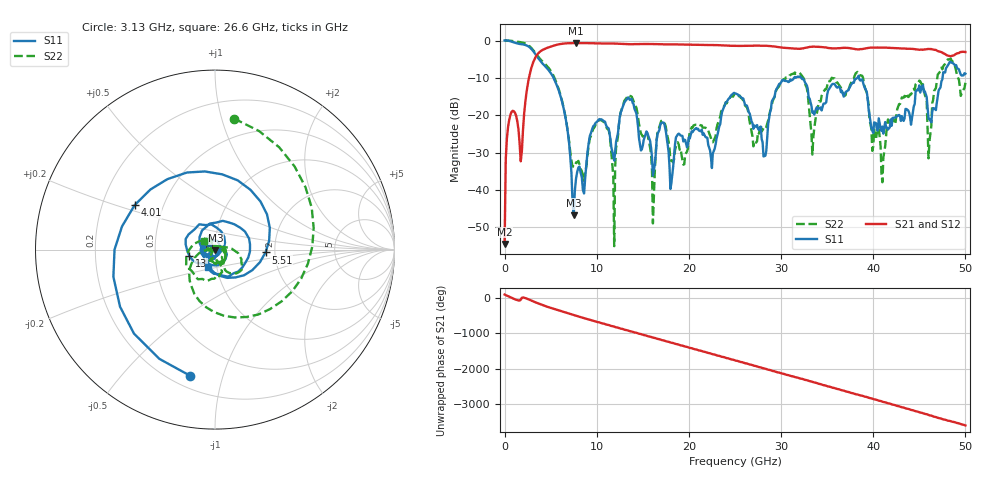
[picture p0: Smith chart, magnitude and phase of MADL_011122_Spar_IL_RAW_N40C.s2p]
#	HZ	S	DB	R	50
!Frequency	S11 (dB)	S11-Ang	S21 (dB)	S21-Ang	S12 (dB)	S12-Ang	S22 (dB)	S22-Ang
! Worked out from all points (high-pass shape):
!   401 points, 10 MHz to 50 GHz, reference 50 ohm
!   highest |S21| = -0.68 dB at 7.76 GHz (marker M1); lowest = -54.4 dB at 10 MHz (marker M2)
!   |S21| within 3 dB of the highest: 3.574 GHz to 47.84 GHz (44.26 GHz wide, 172 % of centre); 48.92 GHz to end of sweep
!   lowest |S11| = -46.7 dB at 7.51 GHz (marker M3), VSWR 1.01, Z = 50.3 - j0.383 ohm
!   |S11| at or under -10 dB: 5.324 GHz to 31.4 GHz (26.08 GHz wide, 142 % of centre); 32.2 GHz to 38.27 GHz (6.071 GHz wide, 17.2 % of centre); 38.46 GHz to 47.52 GHz (9.062 GHz wide, 21.1 % of centre)
!   |S22| runs from -55.0 to 0.0 dB; largest |S21 - S12| = 0.016
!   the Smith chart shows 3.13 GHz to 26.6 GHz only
!   S11 on the Smith chart (normalised r, x): 3.13 GHz: 0.27, -0.79; 4.01 GHz: 0.34, +0.23; 5.51 GHz: 1.78, -0.06; 13 GHz: 0.75, -0.05; 26.6 GHz: 0.91, -0.18
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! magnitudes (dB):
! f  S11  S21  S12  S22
! 10 MHz  0.0  -54.4  -52.8  0.0
! 510 MHz  -0.1  -21.2  -21.2  0.0
! 3.13 GHz  -2.9  -5.7  -5.7  -2.6
! 4.01 GHz  -5.8  -2.7  -2.7  -5.3
! 5.51 GHz  -11.0  -1.2  -1.2  -10.5
! 7.51 GHz  -46.7  -0.7  -0.7  -33.7
! 7.76 GHz  -36.9  -0.7  -0.7  -32.6
! 8.38 GHz  -36.5  -0.7  -0.7  -34.9
! 10.5 GHz  -21.1  -0.8  -0.8  -21.2
! 11.9 GHz  -32.1  -0.8  -0.8  -55.0
! 13 GHz  -16.6  -0.9  -0.9  -16.1
! 16.1 GHz  -36.1  -0.9  -0.9  -48.9
! 16.8 GHz  -23.9  -1.0  -1.0  -23.1
! 22.5 GHz  -34.1  -1.2  -1.2  -27.1
! 25.1 GHz  -14.2  -1.4  -1.4  -15.0
! 26.6 GHz  -19.5  -1.4  -1.4  -21.8
! 31.8 GHz  -9.6  -2.2  -2.2  -8.8
! 33.4 GHz  -19.3  -1.6  -1.6  -30.5
! 38.3 GHz  -9.9  -2.3  -2.3  -8.4
! 41 GHz  -23.0  -1.9  -1.9  -37.9
! 41.8 GHz  -23.2  -2.0  -1.9  -22.2
! 50 GHz  -8.9  -3.1  -3.0  -11.3
